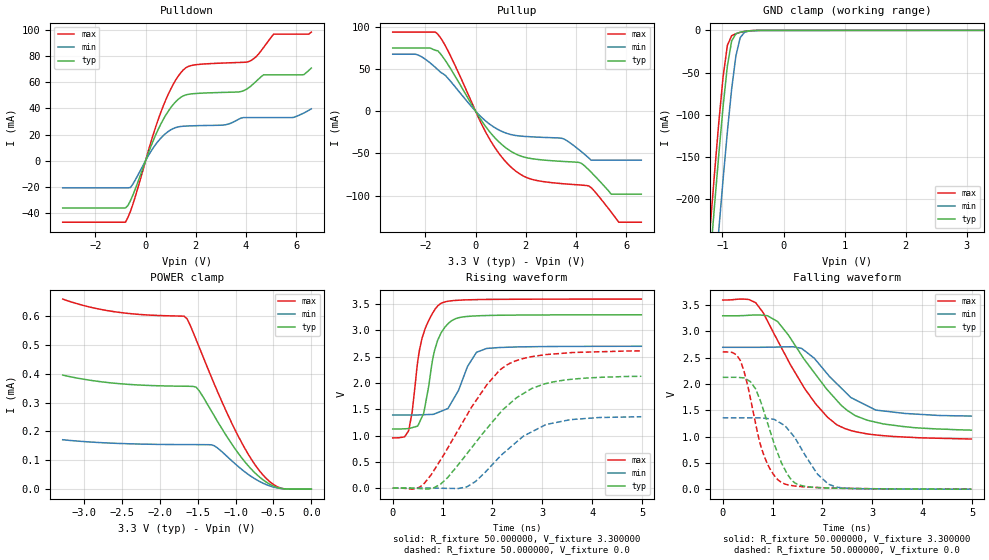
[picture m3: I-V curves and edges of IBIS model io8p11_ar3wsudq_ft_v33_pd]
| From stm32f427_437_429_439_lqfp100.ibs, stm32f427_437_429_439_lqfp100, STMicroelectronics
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|   Model io8p11_ar3wsudq_ft_v33_pd
[Model]  io8p11_ar3wsudq_ft_v33_pd
Model_type I/O
Polarity   Non-Inverting
Enable   Active-Low
Vinl =   0.990000V
Vinh =   2.310000V
Vmeas =  1.650000V
Cref =   30.000000pF
Rref =   100.000000M
Vref =   0.0V
C_comp   3.857500pF   3.760500pF   3.941700pF
[Temperature Range]   25.000000   0.125000k   -40.000000
[Pullup Reference]   3.300000V   2.700000V   3.600000V
[Pulldown Reference]   0.0V   0.0V   0.0V
[POWER Clamp Reference]   3.300000V   2.700000V   3.600000V
[GND Clamp Reference]   0.0V   0.0V   0.0V
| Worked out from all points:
|   slope of the pulldown table from 0 to 0.495 V, typ, clamps not added: 20.9 ohm
|   slope of the pullup table from 0 to 0.495 V, typ, clamps not added: 22.6 ohm
|   GND clamp passes 1 mA (typ) near -0.62 V on its own axis
|   rising waveform, R_fixture 50.000000, V_fixture 3.300000: 20-80 % time 278ps typ, 390ps min, 271ps max; typ from 1.12 V to 3.3 V
|   rising waveform, R_fixture 50.000000, V_fixture 0.0: 20-80 % time 1.16ns typ, 998ps min, 1.05ns max; typ from 0 V to 2.13 V
|   falling waveform, R_fixture 50.000000, V_fixture 3.300000: 20-80 % time 1.06ns typ, 877ps min, 1.03ns max; typ from 3.3 V to 1.12 V
|   falling waveform, R_fixture 50.000000, V_fixture 0.0: 20-80 % time 472ps typ, 561ps min, 409ps max; typ from 2.13 V to 0 V
[Pulldown]
|Voltage   I(typ)   I(min)   I(max)
-3.3V     -36.18mA   -20.77mA   -47.07mA
-800mV    -36.18mA   -20.77mA   -47.07mA
-600mV    -30.5mA    -20.52mA   -38.69mA
700mV     31.4mA     19.11mA    41.71mA
1.2V      45.15mA    25.37mA    61.75mA
1.6V      50.35mA    26.5mA     71.06mA
3.1V      52.27mA    27.26mA    74.75mA
4.1V      55.7mA     32.99mA    75.8mA
4.7V      65.71mA    32.99mA    86.63mA
5.1V      65.71mA    32.99mA    96.88mA
6.3V      65.85mA    36.49mA    96.88mA
6.6V      70.9mA     39.7mA     98.44mA
[Pullup]
|Voltage   I(typ)   I(min)   I(max)
-3.3V     74.74mA    67.41mA    93.59mA
-2.3V     74.74mA    66.57mA    93.59mA
-1.5V     71.35mA    49.01mA    91.01mA
-1V       50.51mA    35.5mA     65.49mA
500mV     -22.07mA   -14mA      -30.03mA
1.6V      -50.64mA   -28.81mA   -70.96mA
3.5V      -59.53mA   -32.72mA   -85.92mA
4.2V      -61.52mA   -47.6mA    -87.46mA
4.5V      -69.21mA   -55.15mA   -88.44mA
5.4V      -98.2mA    -58mA      -119.4mA
5.7V      -98.2mA    -58mA      -131.4mA
6.6V      -98.2mA    -58mA      -131.4mA
[GND_clamp]
|Voltage   I(typ)   I(min)   I(max)
-3.3V     -2.332A    -2.407A    -2.312A
-1.2V     -270.2mA   -361.4mA   -232.1mA
-1.13V    -207.3mA   -298.1mA   -169mA
-1.06V    -146.7mA   -236.2mA   -108.8mA
-990mV    -90.18mA   -176.4mA   -54.97mA
-920mV    -42.21mA   -120mA     -17.69mA
-850mV    -12.58mA   -69.47mA   -6.279mA
-780mV    -3.983mA   -30.01mA   -3.9mA
-710mV    -2.112mA   -8.623mA   -2.396mA
-640mV    -1.159mA   -2.292mA   -1.234mA
-570mV    -535.1uA   -830.5uA   -490.2uA
3.28V     81.28uA    57.87uA    93.98uA
[POWER_clamp]
|Voltage   I(typ)   I(min)   I(max)
-3.28V    395.3uA    171.3uA    658.7uA
-2.6V     367.1uA    159uA      614.9uA
-1.68V    356.7uA    154.4uA    599.4uA
-1.64V    356.5uA    154.4uA    590.8uA
-1.52V    353.6uA    154.3uA    518.3uA
-1.48V    341.1uA    154.2uA    492.3uA
-1.28V    253.6uA    150.4uA    364.2uA
-960mV    123.1uA    77.55uA    181.6uA
-720mV    50.52uA    32.03uA    76.18uA
-560mV    18.94uA    12.27uA    28.65uA
-440mV    5.104uA    3.69uA     7.327uA
0V        0A         0A         0A
[Ramp]
| variable   typ   min   max
dV/dt_r  1.26420/1.15771n   0.80682/0.99254n   1.56096/1.04850n
dV/dt_f  1.28064/1.04421n   0.77262/0.86595n   1.57145/1.02312n
R_load = 50.000000
[Rising Waveform]
R_fixture= 50.000000
V_fixture= 3.300000
V_fixture_min= 2.700000
V_fixture_max= 3.600000
|time   V(typ)   V(min)   V(max)
0s        1.123V     1.391V     953.8mV
320.3ps   1.131V     1.39V      1.094V
510.5ps   1.197V     1.391V     2.471V
650.7ps   1.571V     1.397V     3.037V
830.8ps   2.585V     1.408V     3.377V
971ps     2.955V     1.462V     3.517V
1.111ns   3.13V      1.519V     3.557V
1.682ns   3.278V     2.585V     3.587V
1.882ns   3.284V     2.657V     3.591V
4.985ns   3.299V     2.699V     3.598V
[Rising Waveform]
R_fixture= 50.000000
V_fixture= 0.0
V_fixture_min= 0.0
V_fixture_max= 0.0
|time   V(typ)   V(min)   V(max)
0s        211.7uV    82.57uV    620.3uV
550.6ps   -10.61mV   -118.1uV   23.35mV
951ps     68.5mV     -3.811mV   522.3mV
1.491ns   656.9mV    24.75mV    1.394V
1.882ns   1.125V     327.7mV    1.959V
2.282ns   1.553V     713.1mV    2.34V
2.783ns   1.893V     1.068V     2.501V
3.073ns   1.989V     1.209V     2.541V
3.574ns   2.069V     1.303V     2.578V
4.985ns   2.127V     1.358V     2.61V
[Falling Waveform]
R_fixture= 50.000000
V_fixture= 3.300000
V_fixture_min= 2.700000
V_fixture_max= 3.600000
|time   V(typ)   V(min)   V(max)
0s        3.299V     2.699V     3.598V
660.7ps   3.314V     2.699V     3.548V
810.8ps   3.307V     2.7V       3.359V
1.101ns   3.188V     2.704V     2.828V
1.582ns   2.546V     2.678V     2.012V
1.872ns   2.171V     2.45V      1.614V
2.292ns   1.684V     2.002V     1.224V
2.663ns   1.397V     1.699V     1.094V
3.073ns   1.273V     1.504V     1.031V
4.985ns   1.123V     1.391V     953.8mV
[Falling Waveform]
R_fixture= 50.000000
V_fixture= 0.0
V_fixture_min= 0.0
V_fixture_max= 0.0
|time   V(typ)   V(min)   V(max)
0s        2.127V     1.358V     2.61V
350.4ps   2.123V     1.357V     2.454V
510.5ps   2.072V     1.357V     1.934V
660.7ps   1.907V     1.356V     1.244V
860.9ps   1.372V     1.346V     559.8mV
1.191ns   476.2mV    1.24V      121.1mV
1.491ns   97.47mV    908.2mV    55.7mV
1.902ns   30.43mV    284.2mV    31.08mV
2.282ns   17.95mV    39.13mV    18.7mV
4.985ns   211.7uV    82.57uV    620.3uV
